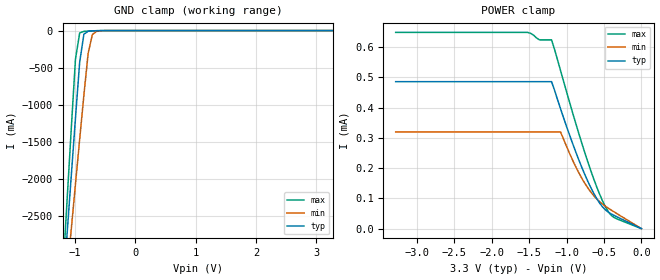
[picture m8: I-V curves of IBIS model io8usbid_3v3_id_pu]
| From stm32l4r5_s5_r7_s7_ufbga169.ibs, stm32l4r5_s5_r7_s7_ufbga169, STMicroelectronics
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|   Model io8usbid_3v3_id_pu
[Model]  io8usbid_3v3_id_pu
Model_type Input
Polarity   Non-Inverting
Vinl =   0.540000V
Vinh =   1.260000V
C_comp   2.116400pF   2.092900pF   2.152900pF
[Temperature Range]   25.000000   0.125000k   -40.000000
[Pullup Reference]   3.300000V   2.700000V   3.600000V
[Pulldown Reference]   0.0V   0.0V   0.0V
[POWER Clamp Reference]   3.300000V   2.700000V   3.600000V
[GND Clamp Reference]   0.0V   0.0V   0.0V
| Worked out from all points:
|   GND clamp passes 1 mA (typ) near -0.59 V on its own axis
[GND_clamp]
|Voltage   I(typ)   I(min)   I(max)
-3.3V     -9.914A    -9.595A    -9.188A
-1.2V     -3.541A    -3.911A    -3.279A
-1.13V    -2.75A     -3.295A    -2.301A
-1.06V    -1.963A    -2.68A     -1.33A
-990mV    -1.183A    -2.069A    -386.7mA
-920mV    -424.7mA   -1.463A    -31.42mA
-850mV    -49.12mA   -868.7mA   -10.48mA
-780mV    -9.121mA   -308.3mA   -6.715mA
-710mV    -3.648mA   -53.81mA   -3.986mA
-640mV    -1.726mA   -11.03mA   -1.885mA
-430mV    -22.46uA   -116.8uA   -9.748uA
3.28V     0A         0A         0A
[POWER_clamp]
|Voltage   I(typ)   I(min)   I(max)
-3.28V    486.2uA    319.9uA    649.2uA
-1.52V    486.2uA    319.9uA    649.2uA
-1.36V    486.2uA    319.9uA    624.4uA
-1.2V     486.2uA    319.9uA    624.4uA
-1.08V    396.5uA    319.9uA    523.1uA
-920mV    282.6uA    227.1uA    384.4uA
-800mV    205.1uA    168.4uA    285.8uA
-640mV    118.3uA    110.1uA    166.6uA
-520mV    72.17uA    81.22uA    92.15uA
-440mV    54.23uA    67.17uA    54.98uA
-400mV    48.29uA    60.81uA    43.12uA
0V        0A         0A         0A
